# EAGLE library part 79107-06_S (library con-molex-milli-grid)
RECEPTACAL
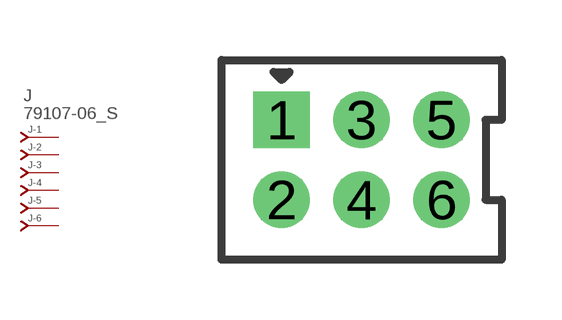
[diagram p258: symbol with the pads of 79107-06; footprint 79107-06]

Designator prefix J; gates -1=J-NV -2=J-N -3=J-N -4=J-N -5=J-N -6=J-N

## 79107-06_S  [79107-06]
1  -1:J  pas
2  -2:J  pas
3  -3:J  pas
4  -4:J  pas
5  -5:J  pas
6  -6:J  pas

## Footprint 79107-06 (pad centres in mm)
RECEPTACAL Dual Row, Vertical, Through-Hole
drill 0.914 square: 1 -2,1
drill 0.914: 2 -2,-1; 3 0,1; 4 0,-1; 5 2,1; 6 2,-1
